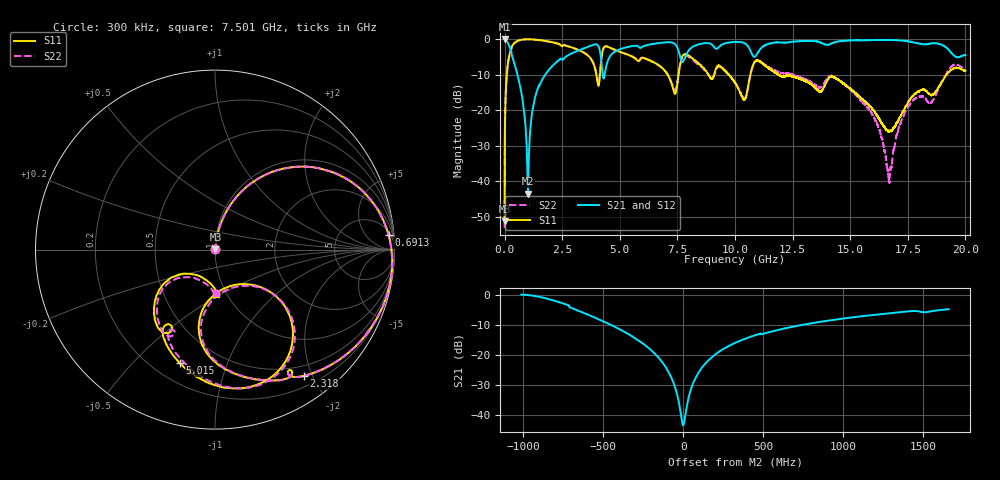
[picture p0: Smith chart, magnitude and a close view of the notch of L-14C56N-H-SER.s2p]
!{L-14C56N}
!Johanson Technology Inc.
!www.johansontechnology.com
!Test Board Conditions:
!Substrate Type  RO4350B
!Substrate Thickness  20 mil
!Substrate Dk  3.66
!TL Type: GCPW
!TL Trace Width  36 mil
!TL Gap  12 mil
!Electrode orientation  Horizontal
!DUT TOPOLOGY	SERIES
!Mounting Pad LxW  26x36 mil
! Created Sun Jun 20 13:06:50 2021
# hz S ma R 50
! 2 Port Network Data from SP1.SP block
! freq  magS11  angS11  magS21  angS21  magS12  angS12  magS22  angS22
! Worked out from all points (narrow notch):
!   20001 points, 300 kHz to 20 GHz, reference 50 ohm
!   highest |S21| = -0.01 dB at 1.3 MHz (marker M1); lowest = -43.6 dB at 1.012 GHz (marker M2)
!   notch at M2: 42.1 dB deep, 277 MHz wide at half that depth
!   lowest |S11| = -51.3 dB at 300 kHz (marker M3), VSWR 1.01, Z = 50.2 + j0.116 ohm
!   |S11| at or under -10 dB: 7.072 GHz to 7.547 GHz (474.6 MHz wide, 6.49 % of centre); 9.73 GHz to 10.67 GHz (940.1 MHz wide, 9.22 % of centre); 11.89 GHz to 19.19 GHz (7.3 GHz wide, 47 % of centre)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
!   |S22| runs from -53.1 to -0.1 dB; largest |S21 - S12| = 0.011
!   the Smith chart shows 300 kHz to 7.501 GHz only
!   S11 on the Smith chart (normalised r, x): 300 kHz: 1.00, +0.00; 691.3 MHz: 8, +21; 2.318 GHz: 0.35, -1.88; 5.015 GHz: 0.31, -0.69; 7.501 GHz: 0.90, -0.47
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300000  0.002734 24.9  0.998 -0.2  0.9975 -0.1  0.002214 27.1
1300000  0.004541 80.3  0.9993 -0.3  0.999 -0.4  0.004735 78.1
1.623e8  0.4921 56.8  0.8513 -31.4  0.8522 -31.3  0.4945 56.5
6.913e8  0.9705 4.8  0.2029 -82.9  0.2027 -82.8  0.9707 4.6
1.0123e9  0.9924 -10.3  0.006636 -9.4  0.006752 -9.9  0.992 -10.6
1.3993e9  0.9747 -25.4  0.1835 62.5  0.1843 62.4  0.9729 -25.8
2.3183e9  0.861 -54.8  0.4933 33.9  0.4933 33.9  0.859 -55.0
3.3343e9  0.6722 -84.7  0.7179 3.7  0.7194 3.7  0.6714 -84.2
4.0483e9  0.2331 -84.3  0.8167 -38.2  0.8168 -38.2  0.2432 -81.6
4.2583e9  0.6852 -51.5  0.3106 -49.2  0.3111 -49.3  0.6933 -50.6
5.0153e9  0.6609 -107.3  0.7208 -18.7  0.7224 -18.4  0.6584 -104.4
6.6673e9  0.4319 -140.1  0.8745 -52.7  0.8764 -52.6  0.4309 -138.0
7.5013e9  0.2469 -88.3  0.7537 -86.9  0.7544 -86.9  0.2451 -88.7
7.8563e9  0.6166 -120.3  0.576 -57.9  0.5794 -57.8  0.5896 -124.1
1.00003e10  0.2422 -171.3  0.9117 -100.8  0.913 -100.8  0.2459 177.9
1.04173e10  0.1404 -139.3  0.8723 -115.2  0.8739 -115.2  0.1451 -149.9
1.07923e10  0.4366 -129.3  0.575 -116.6  0.5779 -116.8  0.4301 -136.3
1.33343e10  0.2275 132.0  0.9384 -141.9  0.9363 -141.8  0.2425 137.4
1.57213e10  0.1239 109.4  0.9631 -174.4  0.9603 -174.4  0.1108 97.6
1.66673e10  0.04965 156.0  0.9688 169.1  0.9695 169.3  0.01155 9.6
1.75943e10  0.1399 -157.0  0.9182 151.4  0.9198 151.3  0.1224 -134.6
2e10  0.3583 128.5  0.5964 128.4  0.5903 128.7  0.3813 124.4
